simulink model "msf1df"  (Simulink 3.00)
settings: Solver=ode45  SolverMode=SingleTasking  StartTime=0.0  StopTime=30  MaxStep=10  RelTol=1e-5  AbsTol=1e-6
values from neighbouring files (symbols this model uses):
  Disturb = Setpoint    [mimo_MSF1DF_sim.m]    (also in mimo_MSF2DF_sim.m)
  K = 1/kpd    [imc2pseucon.m]    (also in imc2pseudo.m)
  Satlb = temp1    [cback.m]    (also in imcmenu.m = str2num(satlbs))
  Satub = temp1    [cback.m]    (also in imcmenu.m = str2num(satubs))
  Setpoint = zeros(1,n)    [mimo_MSF1DF_sim.m]    (also in mimo_MSF2DF_sim.m)
undefined symbols (not defined in the file or in its folder): denFs, denMs, denPd, denPs, Ksp, Md, Mnt, numFs, numPd, numPs
libraries: MIMO_lib x3, simulink3 x2

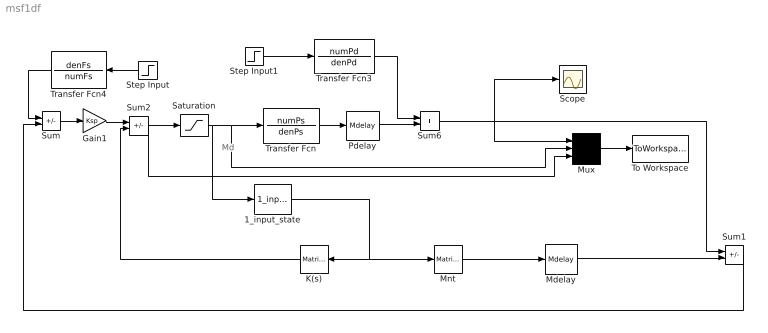
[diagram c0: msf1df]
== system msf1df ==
  note: Md
  1_input_state : MIMO_lib/1_input_state  Ds="[denMs(1)  Md(2:9)]"
  Gain1 : Gain  Gain=Ksp  SaturateOnIntegerOverflow=on
  K(s) : simulink3/Math/Matrix Gain  Orientation=left  K=[0 K(2:9)]
  Mdelay : MIMO_lib/Mdelay  Mdelay=Mdelay
  Mnt : simulink3/Math/Matrix Gain  K=[0 Mnt]
  Mux : Mux  Inputs=3
  Pdelay : MIMO_lib/Mdelay  Mdelay=Pdelay
  Saturation : Saturate  UpperLimit=Satub  LowerLimit=Satlb
  Scope : Scope
  Step Input : Step  Orientation=left  Time=0  Before=0  After=Setpoint  SampleTime=0
  Step Input1 : Step  Time=0  Before=0  After=Disturb  SampleTime=0
  Sum : Sum  Inputs=+-  SaturateOnIntegerOverflow=on
  Sum1 : Sum  Inputs=+-  SaturateOnIntegerOverflow=on
  Sum2 : Sum  Inputs=+-  SaturateOnIntegerOverflow=on
  Sum6 : Sum  Inputs=++  SaturateOnIntegerOverflow=on
  To Workspace : ToWorkspace  VariableName=simout  SampleTime=0  SaveFormat=Matrix
  Transfer Fcn : TransferFcn  Numerator=numPs  Denominator=denPs
  Transfer Fcn3 : TransferFcn  Numerator=numPd  Denominator=denPd
  Transfer Fcn4 : TransferFcn  Orientation=left  Numerator=denFs  Denominator=numFs
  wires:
  Step Input1/1 -> Transfer Fcn3/1
  Transfer Fcn3/1 -> Sum6/1
  Pdelay/1 -> Sum6/2
  Sum2/1 -> Mux/3, Saturation/1
  Mux/1 -> To Workspace/1
  Transfer Fcn/1 -> Pdelay/1
  Gain1/1 -> Sum2/1
  Sum/1 -> Gain1/1
  Sum6/1 -> Mux/1, Sum1/1, Scope/1
  Mnt/1 -> Mdelay/1
  Mdelay/1 -> Sum1/2
  Saturation/1 -> Transfer Fcn/1, Mux/2, 1_input_state/1
  Sum1/1 -> Sum/2
  K(s)/1 -> Sum2/2
  Step Input/1 -> Transfer Fcn4/1
  Transfer Fcn4/1 -> Sum/1
  1_input_state/1 -> K(s)/1, Mnt/1
